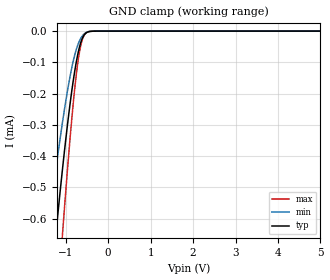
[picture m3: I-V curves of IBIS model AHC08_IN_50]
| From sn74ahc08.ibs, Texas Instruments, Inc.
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[Model]   AHC08_IN_50
Model_type  Input
Vinl=1.65
Vinh=3.9
| variable   typ   min   max
C_comp   0.83pF   0.75pF   0.92pF
[Temperature Range]   40   100   -40
| Ambient temperature   25   85   -40
[Voltage range]   5   4.5   5.5
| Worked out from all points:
|   GND clamp passes 1 mA (typ) near -1.47 V on its own axis
[GND Clamp]
| AHC08_IN_50
|   Voltage   I(typ)   I(min)   I(max)
-5.5V     -8.894mA   -6.578mA   -10.58mA
-1.455V   -977uA     -680.1uA   -1.39mA
-1.4V     -893.9uA   -619.6uA   -1.278mA
-1.23V    -648uA     -440.9uA   -941.7uA
-1.08V    -447.6uA   -296.2uA   -658.7uA
-1.055V   -416.1uA   -273.6uA   -613.2uA
-905mV    -241.4uA   -151uA     -356.2uA
-820mV    -157uA     -94.98uA   -228.2uA
-745mV    -95.21uA   -56.64uA   -133.4uA
-630mV    -30.71uA   -19.84uA   -37.72uA
-510mV    -5.045uA   -3.932uA   -4.663uA
5V        4.223nA    290.1pA    38.48nA
